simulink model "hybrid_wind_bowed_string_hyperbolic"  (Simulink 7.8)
settings: Solver=FixedStepDiscrete  SolverMode=SingleTasking  StartTime=0.0  StopTime=inf  FixedStep=Ts  RelTol=1e-3
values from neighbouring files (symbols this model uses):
  alpha = 0.5    [bowed_string_hyperbolic.m]    (also in polynomial.m = 100)
  amp_gain_factor = 0.73316    [hybrid_wind.m]    (also in measurements.m = 0.73312)
  delta = mu_d/mu_s    (= 0.375)    [bowed_string_hyperbolic.m]
  gammab_cte = 1    [bowed_string_hyperbolic.m]
  HLL_d = c2d(HLL_c,Ts)    [hybrid_wind.m]    (also in measurements.m)
  maxoutputvoltage = 5    [hybrid_wind.m]    (also in measurements.m)
  micoffset_V = mean(voltsin_calib)    [hybrid_wind.m]    (also in measurements.m)
  micpreampsensitivity = -0.0025726    [hybrid_wind.m]    (also in measurements.m)
  PM = 50    [bowed_string_hyperbolic.m]    (also in lip_reed.m = 20; single_reed.m = 100)
  Ts = 25e-6    (= 2.5e-05)    [hybrid_wind.m]    (also in measurements.m)
  Zc = rho*c/St    (= 2615281.00417)    [hybrid_wind.m]
  zetab_cte = 0.2    [bowed_string_hyperbolic.m]
undefined symbols (not defined in the file or in its folder): Bl, cell2mat, Mms, Re, Sd, vibrato
libraries: simulink x5

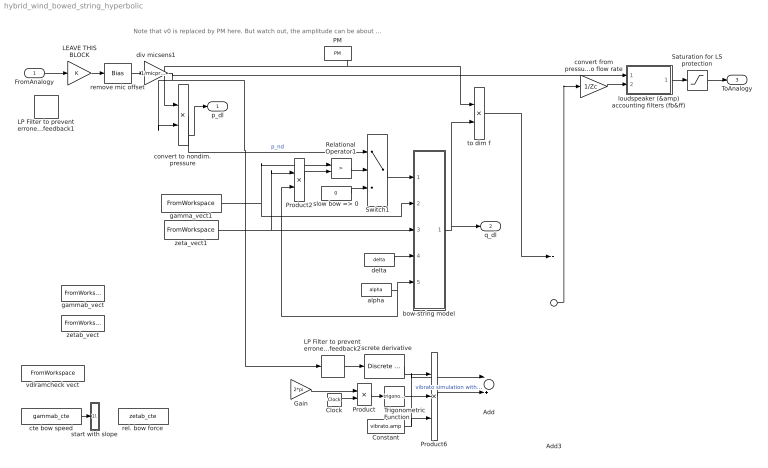
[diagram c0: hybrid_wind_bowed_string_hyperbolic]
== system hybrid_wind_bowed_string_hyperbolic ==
  note: Note that v0 is replaced by PM here. But watch out, the amplitude can be about 8 times higher.
  FromAnalogy : Inport  Interpolate=off
  Add : Sum  Inputs=-+
  Add3 : Sum
  Clock : Clock
  Constant : Constant  Value=vibrato.amp
  Gain : Gain  Gain=2*pi
  LEAVE THIS BLOCK : Gain
  LP Filter to prevent erroneous high freq feedback1 : DiscreteFilter  Numerator=HdLP.ScaleValues(1)*HdLP.sosMatrix(1:end/2)  Denominator=HdLP.ScaleValues(2)*HdLP.sosMatrix(1+end/2:end)  SampleTime=Ts
  LP Filter to prevent erroneous high freq feedback2 : DiscreteFilter  Numerator=HdLP2.ScaleValues(1)*HdLP2.sosMatrix(1:end/2)  Denominator=HdLP2.ScaleValues(2)*HdLP2.sosMatrix(1+end/2:end)  SampleTime=Ts
  PM : Constant  Value=PM
  Product : Product
  Product2 : Product  SampleTime=Ts
  Product6 : Product  Inputs=3
  Relational Operator1 : RelationalOperator  Operator=>  OutDataTypeStr=boolean  SampleTime=Ts
  Saturation for LS protection : Saturate  UpperLimit=maxoutputvoltage  LowerLimit=-maxoutputvoltage
  Switch1 : Switch  Criteria=u2 > Threshold
  Trigonometric Function : Trigonometry
  alpha : Constant  Value=alpha
  bow-string model : Subsystem
  convert from pressure  to flow rate : Gain  Gain=1/Zc
  convert to nondim. pressure : Product  Inputs=/*
  cte bow speed : Constant  Value=gammab_cte
  delta : Constant  Value=delta
  discrete derivative : simulink/Discrete/Discrete Derivative  gainval=1.0  ICPrevScaledInput=0.0  InputProcessing=Inherited  OutMin=[]  OutMax=[]  OutDataType=fixdt(1, 16)  OutScaling=2^-10  DoSatur=off
  div micsens1 : Gain  Gain=1/micpreampsensitivity
  gamma_vect1 : FromWorkspace  VariableName=gammab_envs_all  SampleTime=0
  gammab_vect : FromWorkspace  VariableName=gammab_vect  SampleTime=Ts  OutputAfterFinalValue=Setting to zero
  loudspeaker (&amp) accounting filters (fb&ff) : Subsystem
  rel. bow force : Constant  Value=zetab_cte
  remove mic offset : Bias  Bias=-micoffset_V
  slow bow => 0 : Constant  Value=0
  start with slope : Subsystem
  to dim f : Product
  vdlramcheck vect : FromWorkspace  VariableName=gammabrampcheck_vect  SampleTime=Ts  OutputAfterFinalValue=Setting to zero
  zeta_vect1 : FromWorkspace  VariableName=zetab_envs_all  SampleTime=0  OutputAfterFinalValue=Setting to zero
  zetab_vect : FromWorkspace  VariableName=zetab_vect  SampleTime=Ts  OutputAfterFinalValue=Setting to zero
  p_dl : Outport
  q_dl : Outport  Port=2
  ToAnalogy : Outport  Port=3
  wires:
  PM/1 -> convert to nondim. pressure/1, to dim f/1
  delta/1 -> bow-string model/4(deltab)
  alpha/1 -> bow-string model/5(alpha), Product2/2
  to dim f/1 -> Add3/1
  cte bow speed/1 -> start with slope/1(gamma_in)
  convert to nondim. pressure/1 -> Switch1/1, p_dl/1  "p_nd"
  remove mic offset/1 -> div micsens1/1
  LEAVE THIS BLOCK/1 -> remove mic offset/1
  FromAnalogy/1 -> LEAVE THIS BLOCK/1
  Saturation for LS protection/1 -> ToAnalogy/1
  loudspeaker (&amp) accounting filters (fb&ff)/1(V_amp_in) -> Saturation for LS protection/1
  discrete derivative/1 -> Product6/1
  LP Filter to prevent erroneous high freq feedback2/1 -> discrete derivative/1
  Trigonometric Function/1 -> Product6/2
  Product/1 -> Trigonometric Function/1
  Clock/1 -> Product/2
  Constant/1 -> Product6/3, Add/1
  Product6/1 -> Add/2  "vibrato simulation with variable additional parallel virtual compliance at the entrance"
  Gain/1 -> Product/1
  bow-string model/1(fdl) -> to dim f/2, q_dl/1
  convert from pressure  to flow rate/1 -> loudspeaker (&amp) accounting filters (fb&ff)/2(U_calc)
  div micsens1/1 -> loudspeaker (&amp) accounting filters (fb&ff)/1(P), LP Filter to prevent erroneous high freq feedback2/1, convert to nondim. pressure/2
  zeta_vect1/1 -> bow-string model/3(zetab), Product2/1
  Relational Operator1/1 -> Switch1/2
  Add3/1 -> convert from pressure  to flow rate/1
  slow bow => 0/1 -> Switch1/3
  Switch1/1 -> bow-string model/1(vdl)
  Product2/1 -> Relational Operator1/2
  gamma_vect1/1 -> bow-string model/2(gammab), Relational Operator1/1

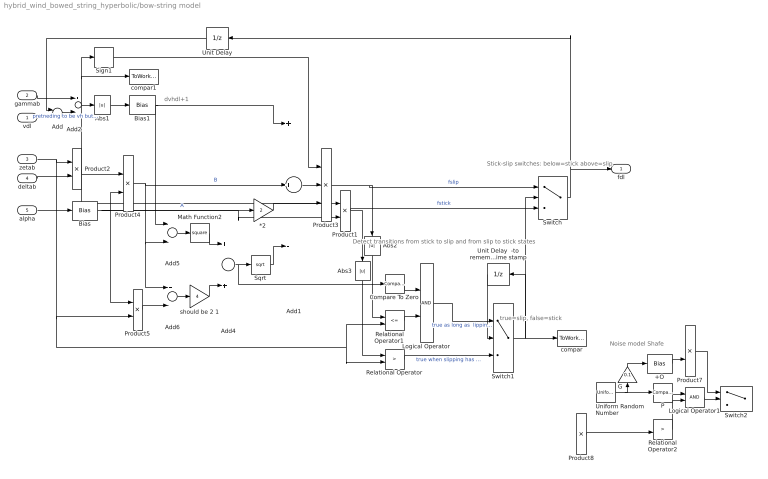
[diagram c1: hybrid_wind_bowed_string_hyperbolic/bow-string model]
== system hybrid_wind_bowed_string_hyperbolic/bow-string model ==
  note: Stick-slip switches: below=stick above=slip
  note: true=slip, false=stick
  note: dvhdl+1
  note: Detect transitions from stick to slip and from slip to stick states
  note: Noise model Shafe
  vdl : Inport
  gammab : Inport  Port=2
  zetab : Inport  Port=3
  deltab : Inport  Port=4
  alpha : Inport  Port=5
  "*2 " : Gain  Gain=2
  +O : Bias  Bias=1
  Abs1 : Abs
  Abs2 : Abs
  Abs3 : Abs
  Add : Sum  Inputs=-+
  Add1 : Sum  Inputs=++-
  Add2 : Sum  Inputs=+-  SampleTime=Ts
  Add4 : Sum
  Add5 : Sum  Inputs=+-
  Add6 : Sum  Inputs=+-
  Bias : Bias  Bias=1
  Bias1 : Bias  Bias=1
  Compare To Zero : simulink/Logic and Bit Operations/Compare To Zero  relop=>  OutDataTypeStr=uint8
  G : Gain  Gain=0.1
  Logical Operator : Logic  AllPortsSameDT=off  OutDataTypeStr=boolean
  Logical Operator1 : Logic  AllPortsSameDT=off  OutDataTypeStr=boolean
  Math Function2 : Math  Operator=square
  P : simulink/Logic and Bit Operations/Compare To Constant  relop=>  const=0.5  OutDataTypeStr=uint8
  Product1 : Product  Inputs=*/
  Product2 : Product  SampleTime=Ts
  Product3 : Product  Inputs=**/
  Product{4..5,7..8} (4 alike) : Product
  Relational Operator : RelationalOperator  Operator=>  OutDataTypeStr=boolean  SampleTime=Ts
  Relational Operator1 : RelationalOperator  Operator=<=  OutDataTypeStr=boolean  SampleTime=Ts
  Relational Operator2 : RelationalOperator  Operator=>  OutDataTypeStr=boolean
  Sign1 : Signum
  Sqrt : Sqrt  OutputSignalType=real
  Switch : Switch  Criteria=u2 > Threshold
  Switch1 : Switch  Criteria=u2 > Threshold
  Switch2 : Switch  Criteria=u2 > Threshold
  Uniform Random Number : UniformRandomNumber  Minimum=0  SampleTime=Ts
  Unit Delay : UnitDelay  SampleTime=-1
  Unit Delay  -to remember slip/stick state of previous time stamp : UnitDelay  SampleTime=-1
  compar : ToWorkspace  VariableName=compar  SampleTime=-1  SaveFormat=Structure
  compar1 : ToWorkspace  VariableName=dvhdl  SampleTime=-1  SaveFormat=Structure
  should be 2 1 : Gain  Gain=4
  fdl : Outport
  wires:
  gammab/1 -> Add2/1
  Switch1/1 -> Unit Delay  -to remember slip/stick state of previous time stamp/1, Switch/2, compar/1
  Unit Delay  -to remember slip/stick state of previous time stamp/1 -> Switch1/2
  Add2/1 -> Sign1/1, compar1/1, Abs1/1, Product1/1
  Relational Operator/1 -> Switch1/3  "true when slipping has to start"
  Unit Delay/1 -> Add/1
  Add/1 -> Add2/2  "pretneding to be vh but is actually vh-1"
  vdl/1 -> Add/2
  Logical Operator/1 -> Switch1/1  "true as long as  lipping is happening"
  zetab/1 -> Product2/1, Product5/2, Relational Operator1/2, Relational Operator/2
  deltab/1 -> Product2/2
  Product2/1 -> Product4/1
  alpha/1 -> Bias/1
  Bias/1 -> "*2 "/1, Product4/2, Product5/1, Product1/2  "A"
  Product4/1 -> Add1/2, Add5/2, Add6/1  "B"
  Bias1/1 -> Add1/1, Add5/1
  Sqrt/1 -> Add1/3
  Add4/1 -> Sqrt/1, Compare To Zero/1
  Math Function2/1 -> Add4/1
  Add6/1 -> should be 2 1/1
  Add5/1 -> Math Function2/1
  should be 2 1/1 -> Add4/2
  Product5/1 -> Add6/2
  Abs1/1 -> Bias1/1
  Sign1/1 -> Product3/1
  Add1/1 -> Product3/2
  "*2 "/1 -> Product3/3
  Product1/1 -> Switch/3, Abs3/1  "fstick"
  Product3/1 -> Switch/1, Abs2/1  "fslip"
  Compare To Zero/1 -> Logical Operator/1
  Relational Operator1/1 -> Logical Operator/2
  Switch/1 -> Unit Delay/1, fdl/1
  Abs2/1 -> Relational Operator1/1
  Abs3/1 -> Relational Operator/1
  Logical Operator1/1 -> Switch2/2
  P/1 -> Logical Operator1/1
  Relational Operator2/1 -> Logical Operator1/2
  Uniform Random Number/1 -> P/1, G/1
  G/1 -> +O/1
  +O/1 -> Product7/2
  Product7/1 -> Switch2/1
  ? -> Relational Operator2/1  "dvhdl"
  Product8/1 -> Relational Operator2/2
  ? -> Product8/1  "1+alpha"
  ? -> Product8/2  "zetab"
  ? -> Product7/1  "fdl in"
  Switch2/1 -> ?  "fdl out"
  ? -> Switch2/3  "fdl in"

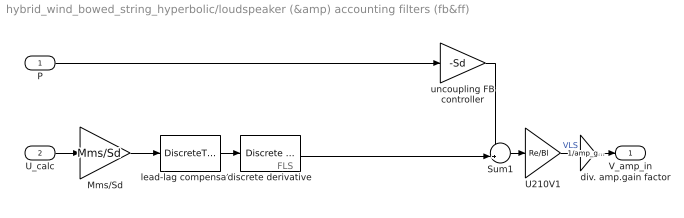
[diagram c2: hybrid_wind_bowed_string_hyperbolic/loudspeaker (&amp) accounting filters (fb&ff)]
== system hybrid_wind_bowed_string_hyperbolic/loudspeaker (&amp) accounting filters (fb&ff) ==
  note: FLS
  P : Inport
  U_calc : Inport  Port=2
  Mms/Sd : Gain  Gain=Mms/Sd
  Sum1 : Sum  Inputs=-+|
  U210V1 : Gain  Gain=Re/Bl
  discrete derivative : simulink/Discrete/Discrete Derivative  gainval=1.0  ICPrevScaledInput=0.0  InputProcessing=Inherited  OutMin=[]  OutMax=[]  OutDataType=fixdt(1, 16)  OutScaling=2^-10  DoSatur=off
  div. amp.gain factor : Gain  Gain=1/amp_gain_factor
  lead-lag compensator : DiscreteTransferFcn  Numerator=cell2mat(HLL_d.num)  Denominator=cell2mat(HLL_d.den)  SampleTime=Ts
  uncoupling FB controller : Gain  Gain=-Sd
  V_amp_in : Outport
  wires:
  Sum1/1 -> U210V1/1
  U210V1/1 -> div. amp.gain factor/1  "VLS"
  U_calc/1 -> Mms/Sd/1
  discrete derivative/1 -> Sum1/2
  uncoupling FB controller/1 -> Sum1/1
  div. amp.gain factor/1 -> V_amp_in/1
  P/1 -> uncoupling FB controller/1
  Mms/Sd/1 -> lead-lag compensator/1
  lead-lag compensator/1 -> discrete derivative/1

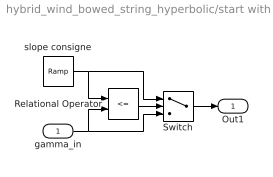
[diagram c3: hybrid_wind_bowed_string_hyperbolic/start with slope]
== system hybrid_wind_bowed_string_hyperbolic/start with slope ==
  gamma_in : Inport
  Relational Operator : RelationalOperator  Operator=<=  OutDataTypeStr=boolean
  Switch : Switch  Criteria=u2 > Threshold
  slope consigne : simulink/Sources/Ramp  slope=gammab_cte*100  start=0  X0=0
  Out1 : Outport
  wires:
  slope consigne/1 -> Relational Operator/1, Switch/1
  gamma_in/1 -> Relational Operator/2, Switch/3
  Relational Operator/1 -> Switch/2
  Switch/1 -> Out1/1
